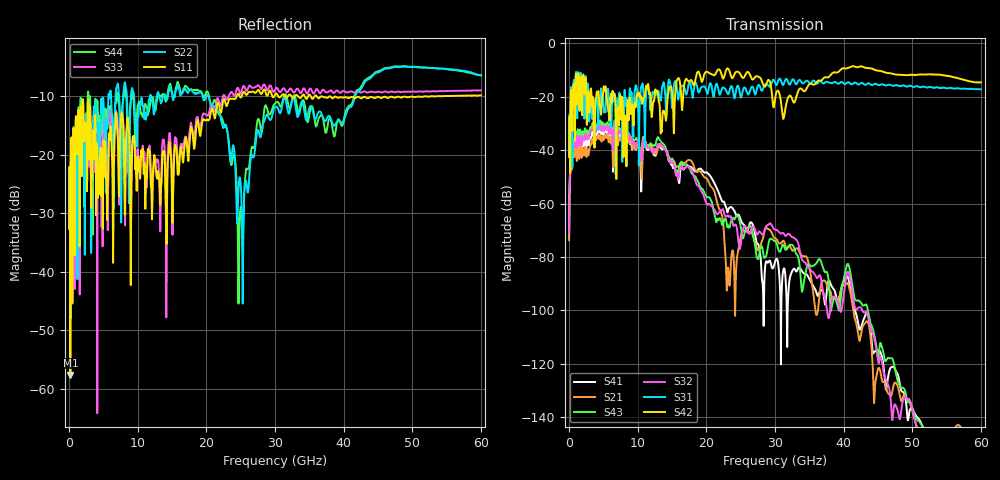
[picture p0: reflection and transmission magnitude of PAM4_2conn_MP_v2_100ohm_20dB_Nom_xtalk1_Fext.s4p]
! Info: Touchstone file created by Circ.  Input file=FAB50GbE_2conn_Midplane_Examax_Topo2_v2_100ohm_20dB_Nom.circ
# Hz S RI R 50
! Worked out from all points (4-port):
!   6000 points, 10 MHz to 60 GHz, reference 50 ohm
!   strongest paths, dB at 10 MHz, 15.01 GHz, 30.01 GHz, 45.01 GHz, 60 GHz:
!     S42: -42.6, -18.4, -20.8, -10.2, -14.6
!     S31: -42.1, -24.2, -14.5, -15.6, -17.2
!     S32: -71.3, -44.1, -69.6, -118.6, -154.2
!     S43: -71.9, -43.7, -74.0, -118.2, -154.5
!     S21: -73.7, -43.1, -72.9, -121.8, -148.5
!     S41: -68.8, -45.4, -81.7, -115.2, -152.2
!   lowest |S11| = -57.6 dB at 190 MHz (marker M1), VSWR 1.00, Z = 50 - j0.131 ohm
!   |S11| at or under -10 dB: start of sweep to 24.4 GHz; 36.9 GHz to 37.89 GHz (989.1 MHz wide, 2.64 % of centre); 38.09 GHz to 50.79 GHz (12.7 GHz wide, 28.6 % of centre)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
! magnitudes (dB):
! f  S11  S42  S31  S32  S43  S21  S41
! 10 MHz  -32.5  -42.6  -42.1  -71.3  -71.9  -73.7  -68.8
! 190 MHz  -57.6  -29.7  -28.5  -45.9  -43.6  -48.4  -45.9
! 6.83 GHz  -12.9  -28.4  -31.4  -33.6  -31.3  -36.8  -33.9
! 17.78 GHz  -15.2  -13.7  -16.5  -47.3  -48.3  -43.9  -46.2
! 23.09 GHz  -11.3  -9.3  -18.8  -64.4  -68.2  -85.3  -63.1
! 24.87 GHz  -10.0  -11.1  -18.4  -77.0  -66.8  -74.1  -65.1
! 60 GHz  -9.8  -14.6  -17.2  -154.2  -154.5  -148.5  -152.2
